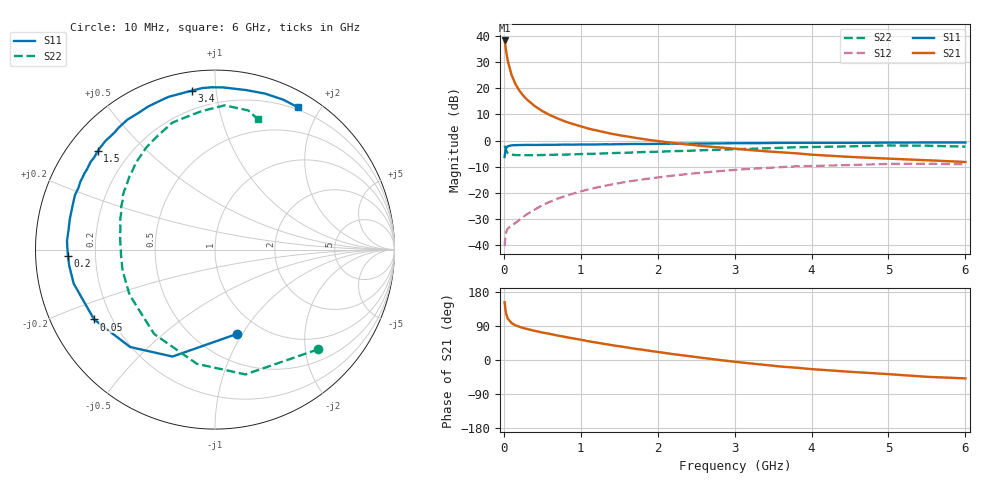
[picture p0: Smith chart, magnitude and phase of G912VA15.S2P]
! SIEMENS Small Signal Semiconductors
! BFG235
! Si NPN RF Bipolar Junction Transistor in SOT223
! VCE = 12 V  IC = 150 mA
! Common Emitter S-Parameters:  July  1994
# GHz  S  MA  R  50
!  f  S11  S21  S12  S22
! GHz  MAG  ANG  MAG  ANG  MAG  ANG  MAG  ANG
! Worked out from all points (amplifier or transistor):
!   40 points, 10 MHz to 6 GHz, reference 50 ohm
!   highest |S21| = 38.3 dB at 10 MHz (marker M1)
!   |S21| within 3 dB of that: start of sweep to 24.51 MHz
!   unconditionally stable (mu >= 1): 457.3 MHz to 1.502 GHz
!   at 200 MHz: K = 0.79, MSG = 24.8 dB, |S12| = -30.4 dB
!   at 1.5 GHz: K = 1.00, MAG = 9.1 dB, |S12| = -16.3 dB
!   at 6 GHz: K = 0.90, MSG = 0.4 dB, |S12| = -9.1 dB
!   S11 on the Smith chart (normalised r, x): 10 MHz: 0.77, -0.95; 50 MHz: 0.13, -0.26; 200 MHz: 0.10, -0.02; 1.5 GHz: 0.09, +0.36; 3.4 GHz: 0.10, +0.86; 6 GHz: 0.17, +1.73
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0.01  0.4856 -75.5  82.6 152.6  0.0095 61.6  0.7996 -44.0
0.02  0.6413 -111.7  65.13 133.9  0.0149 48.4  0.7158 -76.3
0.03  0.72 -131.1  51.28 122.1  0.0177 40.1  0.6444 -99.0
0.05  0.7778 -150.0  34.23 109.5  0.0206 33.5  0.5797 -125.8
0.1  0.8099 -166.5  18.11 97.5  0.0234 35.7  0.5385 -152.1
0.15  0.8172 -173.7  12.16 91.5  0.0264 41.5  0.5273 -163.0
0.2  0.8201 -177.5  9.098 87.8  0.0301 46.8  0.5269 -168.9
0.25  0.8227 179.3  7.328 84.5  0.0343 50.0  0.5237 -172.8
0.3  0.826 176.7  6.119 82.0  0.0388 53.6  0.5246 -176.1
0.4  0.8233 172.3  4.598 77.0  0.0476 57.1  0.5249 179.6
0.5  0.8266 168.3  3.674 72.6  0.0577 58.9  0.5284 176.2
0.6  0.8278 165.2  3.069 68.8  0.0674 59.4  0.5325 173.1
0.7  0.8323 161.6  2.643 64.5  0.0771 59.6  0.5366 170.3
0.9  0.8349 155.9  2.071 57.0  0.0965 57.7  0.5445 165.8
1.1  0.842 149.8  1.696 49.4  0.116 55.4  0.5562 161.2
1.5  0.8532 140.1  1.267 36.2  0.1532 49.2  0.5806 153.0
2.2  0.8732 124.0  0.902 15.5  0.2132 36.8  0.6269 139.6
3.2  0.8897 102.7  0.659 -8.9  0.2866 17.6  0.6953 120.9
3.4  0.8951 98.4  0.624 -13.0  0.2982 13.6  0.7105 116.5
4.5  0.9055 79.0  0.486 -31.1  0.3401 -7.4  0.7747 95.6
5.5  0.9178 65.6  0.42 -44.4  0.3611 -25.8  0.7972 76.6
6  0.9177 59.8  0.389 -48.5  0.3509 -32.6  0.7652 71.8
